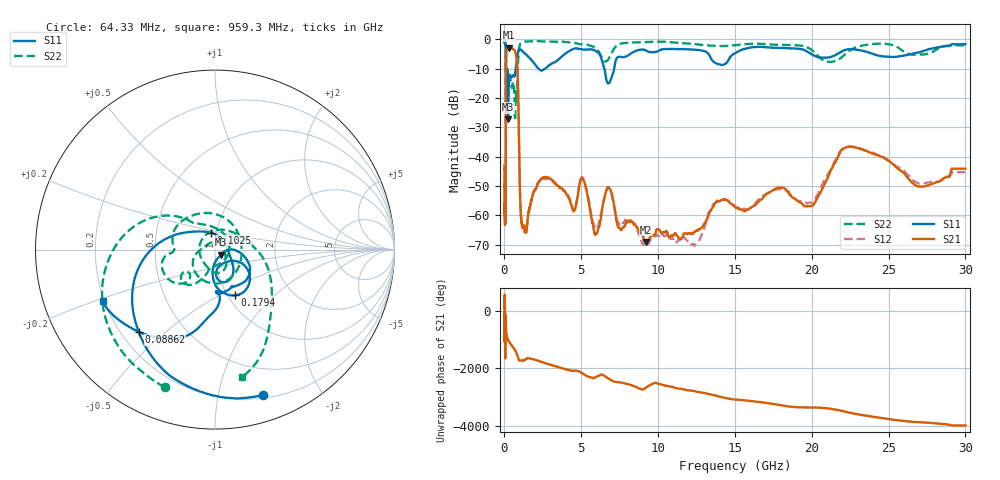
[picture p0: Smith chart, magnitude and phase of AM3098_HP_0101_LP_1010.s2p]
! Date/Time: Thu, Feb 28, 2019 8:36 AM
! Network Analyzer: Agilent Technologies E8364B Rev: A.07.50.67
! Sweep from 0.010 to 30.000 GHz, 1601 Points, Sweep Type: LOG
! Power Supply: 5.022 V, 0.002 A
# Hz S DB R 50
!freq MagS11 AngS11 MagS21 AngS21 MagS12 AngS12 MagS22 AngS22
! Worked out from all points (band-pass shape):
!   1601 points, 10 MHz to 30 GHz, reference 50 ohm
!   highest |S21| = -2.81 dB at 265.1 MHz (marker M1); lowest = -69.1 dB at 9.21 GHz (marker M2)
!   |S21| within 3 dB of the highest: 114.3 MHz to 772.5 MHz (658.2 MHz wide, 148 % of centre)
!   lowest |S11| = -27.2 dB at 237.5 MHz (marker M3), VSWR 1.09, Z = 53.3 - j3.03 ohm
!   |S11| at or under -10 dB: 97.45 MHz to 730.9 MHz (633.4 MHz wide, 153 % of centre); 2.222 GHz to 2.651 GHz (428.4 MHz wide, 17.6 % of centre); 6.506 GHz to 7.139 GHz (633.4 MHz wide, 9.28 % of centre)
!   |S22| runs from -27.7 to -0.6 dB; largest |S21 - S12| = 0.013
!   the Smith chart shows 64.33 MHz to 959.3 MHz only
!   S11 on the Smith chart (normalised r, x): 64.33 MHz: 0.23, -1.36; 88.62 MHz: 0.27, -0.41; 102.5 MHz: 0.94, +0.18; 179.4 MHz: 1.08, -0.60; 959.3 MHz: 0.19, -0.21
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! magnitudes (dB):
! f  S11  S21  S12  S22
! 10 MHz  -0.4  -44.2  -44.1  -0.6
! 38.04 MHz  -0.5  -62.1  -59.3  -0.9
! 64.33 MHz  -1.4  -52.0  -52.6  -1.8
! 79.78 MHz  -2.3  -53.1  -49.6  -2.8
! 88.62 MHz  -4.1  -36.0  -36.0  -4.5
! 102.5 MHz  -20.2  -10.9  -10.9  -21.9
! 144.7 MHz  -17.6  -3.7  -3.6  -13.8
! 179.4 MHz  -11.1  -3.4  -3.3  -10.1
! 237.5 MHz  -27.2  -2.9  -2.9  -12.5
! 265.1 MHz  -18.5  -2.8  -2.8  -12.9
! 550.5 MHz  -12.2  -3.3  -3.2  -14.6
! 825.6 MHz  -6.3  -8.5  -8.5  -17.9
! 959.3 MHz  -3.2  -38.8  -38.9  -2.8
! 1.196 GHz  -4.2  -64.0  -63.9  -0.9
! 2.084 GHz  -9.2  -50.4  -50.0  -0.6
! 5.077 GHz  -3.4  -47.4  -47.0  -1.7
! 5.9 GHz  -3.8  -66.7  -64.3  -2.8
! 7.926 GHz  -5.8  -61.8  -61.8  -1.2
! 9.21 GHz  -3.8  -69.1  -70.2  -0.9
! 19.8 GHz  -4.5  -56.8  -55.7  -3.0
! 22.67 GHz  -3.4  -36.7  -36.6  -3.2
! 30 GHz  -1.6  -44.1  -45.3  -2.0
